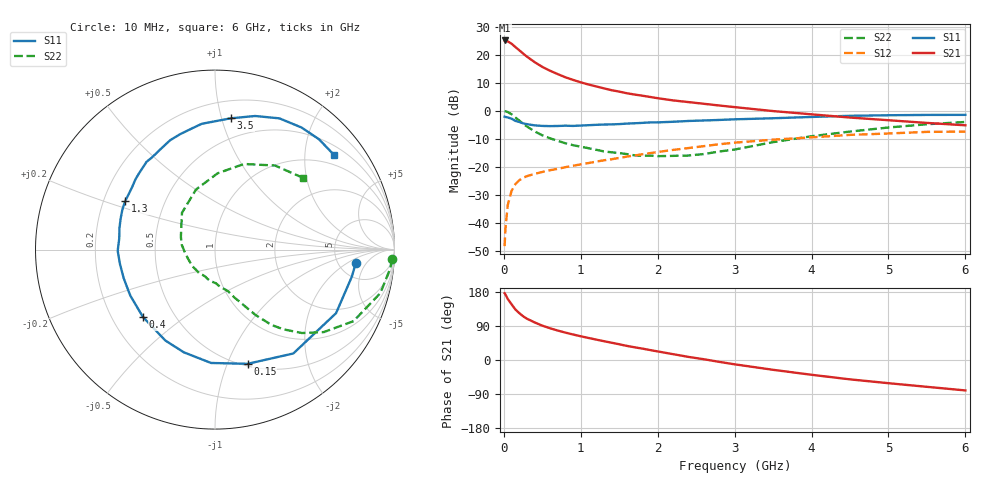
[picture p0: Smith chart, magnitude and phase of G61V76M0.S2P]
! SIEMENS Small Signal Semiconductors
! BFG193
! Si NPN RF Bipolar Junction Transistor in SOT223
! VCE = 1.75 V  IC = 6 mA
! Common Emitter S-Parameters:  August  1996
# GHz  S  MA  R  50
!  f  S11  S21  S12  S22
! GHz  MAG  ANG  MAG  ANG  MAG  ANG  MAG  ANG
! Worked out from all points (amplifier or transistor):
!   36 points, 10 MHz to 6 GHz, reference 50 ohm
!   highest |S21| = 25.2 dB at 10 MHz (marker M1)
!   |S21| within 3 dB of that: start of sweep to 178.4 MHz
!   unconditionally stable (mu >= 1): 1.036 GHz to 2.721 GHz
!   at 250 MHz: K = 0.39, MSG = 22.2 dB, |S12| = -23.9 dB
!   at 1.4 GHz: K = 1.09, MAG = 10.5 dB, |S12| = -17.3 dB
!   at 6 GHz: K = 0.92, MSG = 1.1 dB, |S12| = -7.4 dB
!   S11 on the Smith chart (normalised r, x): 10 MHz: 7.21, -2.91; 150 MHz: 0.52, -1.18; 400 MHz: 0.33, -0.36; 1.3 GHz: 0.29, +0.23; 3.5 GHz: 0.33, +1.07; 6 GHz: 0.72, +2.69
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0.01  0.7873 -5.6  18.13 176.2  0.0038 90.1  0.9877 -3.0
0.02  0.7772 -11.2  18.06 173.3  0.0076 82.1  0.9826 -6.0
0.05  0.7618 -27.7  17.47 161.4  0.0204 75.7  0.9529 -14.7
0.1  0.7248 -53.0  15.89 147.1  0.0369 65.4  0.8689 -27.3
0.15  0.6617 -74.1  13.83 133.3  0.0489 55.9  0.7603 -37.2
0.2  0.632 -92.0  12.13 123.9  0.0573 50.6  0.6715 -43.8
0.25  0.598 -106.9  10.59 115.5  0.0635 46.1  0.5863 -49.3
0.3  0.5771 -118.7  9.317 109.0  0.0678 43.5  0.5255 -53.1
0.4  0.5495 -137.0  7.431 99.2  0.0746 40.7  0.4288 -58.2
0.5  0.537 -151.5  6.11 90.6  0.0805 38.7  0.3652 -61.6
0.6  0.5332 -162.6  5.217 83.8  0.0867 38.7  0.3226 -64.6
0.7  0.5357 -171.6  4.537 77.7  0.0918 38.9  0.2905 -67.7
0.9  0.5371 173.5  3.572 67.3  0.1042 38.9  0.2428 -72.6
1.1  0.5533 161.8  2.956 58.2  0.1163 38.8  0.2147 -80.5
1.3  0.5686 151.7  2.524 49.6  0.1303 38.2  0.1881 -88.2
1.6  0.5912 138.6  2.061 37.2  0.1519 35.9  0.1684 -104.4
2.2  0.6373 118.2  1.536 15.4  0.2 28.5  0.1566 -144.4
2.8  0.6871 100.8  1.245 -4.9  0.2526 18.0  0.1871 171.8
3.5  0.7366 83.2  0.99 -25.9  0.3051 2.4  0.2755 131.9
4.5  0.8144 63.9  0.758 -51.1  0.3713 -17.4  0.4256 88.0
5.5  0.8448 46.7  0.608 -70.8  0.4203 -41.6  0.5754 54.5
6  0.8471 38.6  0.551 -80.3  0.4248 -55.5  0.6321 39.3
